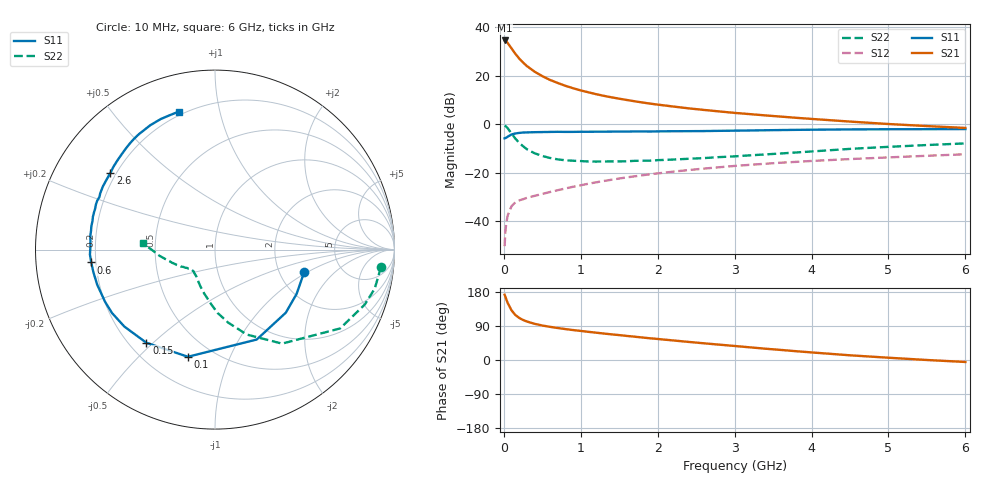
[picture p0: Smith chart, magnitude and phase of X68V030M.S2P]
! SIEMENS Small Signal Semiconductors
! BFP193W
! Si NPN RF Bipolar Junction Transistor in SOT343
! VCE = 8 V  IC = 30 mA
! Common Emitter S-Parameters:  April 1994
# GHz  S  MA  R  50
!  f  S11  S21  S12  S22
! GHz  MAG  ANG  MAG  ANG  MAG  ANG  MAG  ANG
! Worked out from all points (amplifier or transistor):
!   40 points, 10 MHz to 6 GHz, reference 50 ohm
!   highest |S21| = 34.4 dB at 10 MHz (marker M1)
!   |S21| within 3 dB of that: start of sweep to 93.92 MHz
!   unconditionally stable (mu >= 1): 868.2 MHz to 4.435 GHz
!   at 200 MHz: K = 0.42, MSG = 29.2 dB, |S12| = -31.3 dB
!   at 1.5 GHz: K = 1.10, MAG = 14.5 dB, |S12| = -22.3 dB
!   at 6 GHz: K = 0.96, MSG = 5.4 dB, |S12| = -12.4 dB
!   lowest NFmin = 1.90 dB at 450 MHz
!   S11 on the Smith chart (normalised r, x): 10 MHz: 2.76, -0.92; 100 MHz: 0.37, -0.71; 150 MHz: 0.27, -0.48; 600 MHz: 0.18, -0.05; 2.6 GHz: 0.18, +0.32; 6 GHz: 0.18, +0.75
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0.01  0.5127 -13.9  52.77 172.3  0.0031 82.8  0.9302 -5.9
0.02  0.5175 -28.6  52.02 167.1  0.0062 78.8  0.9162 -13.7
0.03  0.5284 -41.7  50.69 161.4  0.0088 75.1  0.8891 -20.1
0.05  0.5523 -65.1  46.78 150.6  0.0133 65.3  0.8241 -32.2
0.1  0.6159 -104.2  36.22 131.1  0.0206 51.4  0.6435 -54.5
0.15  0.6447 -126.4  28.06 118.7  0.0248 45.1  0.5052 -69.5
0.2  0.6625 -139.7  22.35 111.0  0.0271 41.9  0.413 -79.8
0.25  0.6739 -148.4  18.55 105.6  0.0287 41.3  0.3528 -87.7
0.3  0.678 -154.6  15.69 101.6  0.0306 41.8  0.3057 -93.9
0.4  0.6849 -163.5  12.03 95.5  0.0336 43.6  0.2524 -103.7
0.5  0.6893 -169.6  9.732 91.0  0.0368 46.0  0.2221 -111.2
0.6  0.6933 -174.1  8.148 87.5  0.0403 48.1  0.202 -117.1
0.8  0.6944 179.0  6.164 81.6  0.0477 51.7  0.1812 -125.3
1.1  0.6986 171.4  4.527 74.3  0.0597 54.7  0.1709 -133.4
1.3  0.7008 166.9  3.832 69.8  0.0679 56.0  0.171 -136.6
1.6  0.7057 161.1  3.145 63.5  0.0806 56.4  0.1728 -140.3
2.2  0.717 150.5  2.312 51.6  0.1056 54.8  0.1873 -147.2
2.6  0.7225 143.8  1.966 44.1  0.1221 52.8  0.2009 -151.4
3.2  0.7426 134.7  1.61 33.4  0.1461 49.0  0.2288 -158.0
4.5  0.7812 117.5  1.132 12.4  0.1917 40.3  0.3108 -173.6
5.5  0.7898 108.9  0.915 0.0  0.2242 34.1  0.3728 178.0
6  0.795 104.8  0.838 -5.2  0.241 31.4  0.4028 174.9
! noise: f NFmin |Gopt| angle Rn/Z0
0.45  1.9  0.4  180  0.09
0.9  1.95  0.43  -173  0.11
1.8  2.4  0.58  -144  0.24
